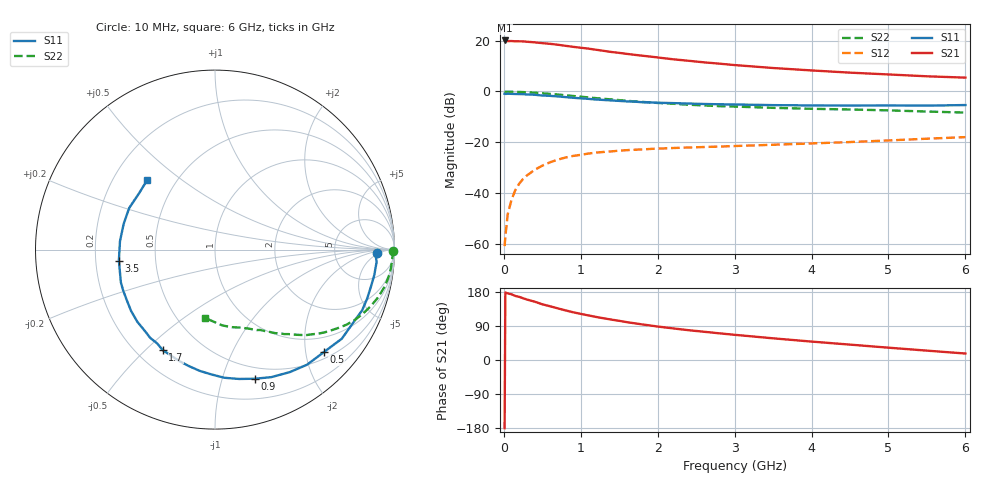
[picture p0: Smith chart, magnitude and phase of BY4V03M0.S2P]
! SIEMENS Small Signal Semiconductors
! BFY420
! Si NPN RF SIEGET Grounded Emitter Transistor in MICRO-X
! VCE = 4 V  IC = 3 mA
! Common Emitter S-Parameters:  October  1996
# GHz  S  MA  R  50
!  f  S11  S21  S12  S22
! GHz  MAG  ANG  MAG  ANG  MAG  ANG  MAG  ANG
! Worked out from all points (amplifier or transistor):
!   36 points, 10 MHz to 6 GHz, reference 50 ohm
!   highest |S21| = 20.1 dB at 10 MHz (marker M1)
!   |S21| within 3 dB of that: start of sweep to 1.037 GHz
!   unconditionally stable (mu >= 1): 3.644 GHz to end of sweep
!   at 250 MHz: K = 0.09, MSG = 27.1 dB, |S12| = -34.4 dB
!   at 1.4 GHz: K = 0.38, MSG = 19.6 dB, |S12| = -23.6 dB
!   at 6 GHz: K = 1.18, MAG = 9.1 dB, |S12| = -18.0 dB
!   S11 on the Smith chart (normalised r, x): 10 MHz: 19, -3; 500 MHz: 0.63, -2.37; 900 MHz: 0.39, -1.28; 1.7 GHz: 0.30, -0.57; 3.5 GHz: 0.30, -0.05; 6 GHz: 0.35, +0.38
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0.01  0.9021 -1.1  10.12 -180.0  0.0009 46.5  0.9906 -0.5
0.02  0.8953 -1.9  10.02 178.1  0.0014 60.4  0.9844 -0.8
0.05  0.903 -4.4  9.827 175.8  0.0038 80.2  0.9905 -2.0
0.1  0.8987 -9.1  9.852 173.4  0.0074 83.7  0.9873 -4.2
0.15  0.893 -13.4  9.738 169.0  0.0115 77.3  0.9852 -6.4
0.2  0.8906 -17.9  9.734 166.6  0.0153 77.2  0.9808 -8.3
0.25  0.8868 -22.4  9.699 162.9  0.019 76.1  0.9736 -10.5
0.3  0.8742 -26.5  9.547 159.6  0.0222 74.7  0.9664 -12.5
0.4  0.8635 -35.1  9.277 154.0  0.0286 69.5  0.9465 -16.4
0.5  0.8329 -43.4  8.951 147.0  0.0347 66.0  0.9228 -20.0
0.7  0.7997 -58.6  8.338 136.3  0.0455 58.6  0.872 -26.7
0.9  0.7527 -72.9  7.577 126.0  0.0538 51.8  0.8165 -32.2
1.1  0.7158 -85.9  6.983 117.6  0.06 46.6  0.7647 -37.1
1.4  0.6657 -102.4  5.99 106.5  0.0662 40.8  0.698 -43.0
1.7  0.6315 -117.4  5.279 96.9  0.0713 36.6  0.6382 -47.7
2  0.5997 -130.2  4.68 88.3  0.0749 33.4  0.5945 -51.8
2.2  0.5906 -137.1  4.307 83.4  0.0771 31.8  0.5738 -54.2
2.8  0.5604 -155.8  3.537 70.4  0.0824 29.0  0.514 -60.6
3.5  0.539 -173.5  2.9 57.2  0.0894 27.4  0.4765 -67.3
4.5  0.5286 164.3  2.351 40.6  0.1011 25.8  0.4422 -77.7
5.5  0.5267 143.5  1.992 24.7  0.1176 23.3  0.4029 -90.7
6  0.5411 134.3  1.875 17.1  0.1263 21.6  0.3844 -98.3
